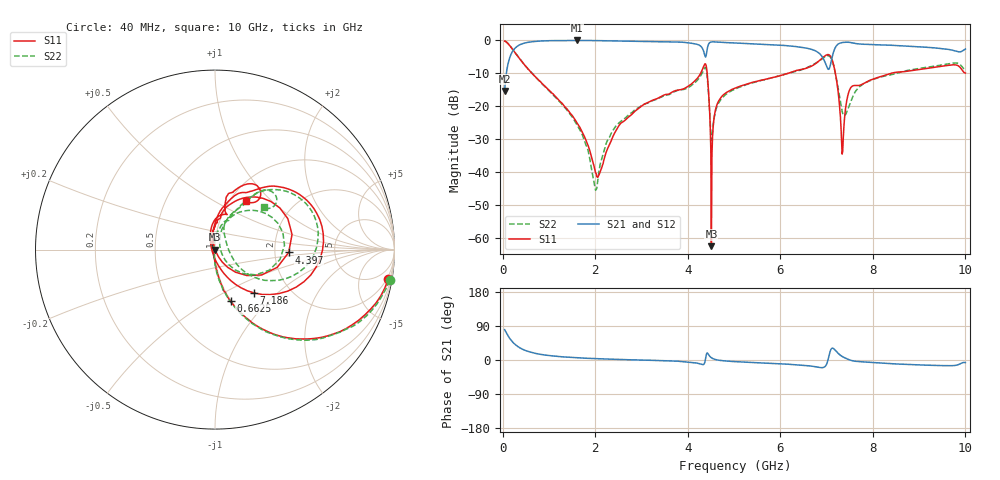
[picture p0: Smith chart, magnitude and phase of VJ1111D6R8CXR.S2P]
! VJ1111D6R8CXR
! DATE 03/04/2022  14:20
! CAPACITORS MOUNTED IN SERIES ON 25 MIL THICK MICROSTRIP SUBSTRATE
# GHz  S  MA  R  50.00
!  FREQ  S11M  S11A  S21M  S21A  S12M  S12A  S22M  S22A
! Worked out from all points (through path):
!   801 points, 40 MHz to 10 GHz, reference 50 ohm
!   highest |S21| = 0.00 dB at 1.596 GHz (marker M1); lowest = -15.4 dB at 40 MHz (marker M2)
!   group delay of S21, straight-line fit = 9.27 ps
!   lowest |S11| = -62.6 dB at 4.51 GHz (marker M3), VSWR 1.00, Z = 50.1 + j0.0243 ohm
!   |S11| at or under -10 dB: 632.3 MHz to 4.277 GHz (3.645 GHz wide, 148 % of centre); 4.418 GHz to 6.168 GHz (1.75 GHz wide, 33.1 % of centre); 7.19 GHz to 8.394 GHz (1.204 GHz wide, 15.5 % of centre)
!   |S22| runs from -45.6 to -0.1 dB; largest |S21 - S12| = 0.011
!   S11 on the Smith chart (normalised r, x): 40 MHz: 2, -12; 662.5 MHz: 0.99, -0.63; 4.397 GHz: 2.39, -0.09; 7.186 GHz: 1.34, -0.72; 10 GHz: 1.18, +0.71
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0.04  0.9778 -9.7  0.1701 80.1  0.1708 79.5  0.9875 -10.0
0.22675  0.7109 -44.5  0.7073 45.6  0.7075 46.3  0.716 -44.9
0.6625  0.3011 -73.2  0.9613 18.6  0.9646 18.6  0.2999 -73.7
1.59625  0.05685 -92.8  1 5.9  1.004 5.8  0.05307 -93.7
1.7083  0.04154 -95.7  0.9989 5.2  1.004 5.1  0.03774 -96.4
2.0071  0.009573 -139.7  0.9953 3.5  0.9992 3.4  0.005241 179.8
2.4055  0.03751 114.8  0.9826 1.9  0.9869 1.7  0.04566 91.4
3.36415  0.1332 89.8  0.9549 -1.5  0.9592 -1.6  0.1309 76.6
4.2979  0.3385 59.1  0.7918 -11.4  0.7948 -11.6  0.3065 45.5
4.3975  0.411 -2.2  0.5939 12.9  0.5965 12.8  0.3658 -8.7
4.50955  0.0007391 19.1  0.9497 6.0  0.9537 5.9  0.0301 6.6
4.5469  0.04765 101.7  0.9527 3.4  0.9572 3.2  0.05095 59.1
4.58425  0.07883 98.7  0.9502 1.7  0.9547 1.6  0.07511 68.3
4.65895  0.117 94.0  0.9438 -0.3  0.9474 -0.5  0.109 70.8
5.02  0.1879 85.2  0.9148 -4.3  0.9187 -4.4  0.1816 67.4
6.6883  0.411 55.0  0.7267 -16.5  0.73 -16.6  0.4209 50.8
7.0369  0.6094 8.4  0.3634 3.5  0.3648 3.3  0.5852 12.3
7.1863  0.3256 -47.9  0.7765 25.8  0.7798 25.6  0.3254 -31.7
7.34815  0.0206 161.4  0.9313 8.5  0.9351 8.5  0.07742 -3.4
7.5349  0.1962 79.6  0.9255 -1.2  0.9297 -1.4  0.1238 66.5
8.34415  0.3076 77.4  0.8474 -9.3  0.8523 -9.4  0.2959 57.4
10  0.319 57.6  0.7409 -6.9  0.7443 -7.1  0.3596 41.2
